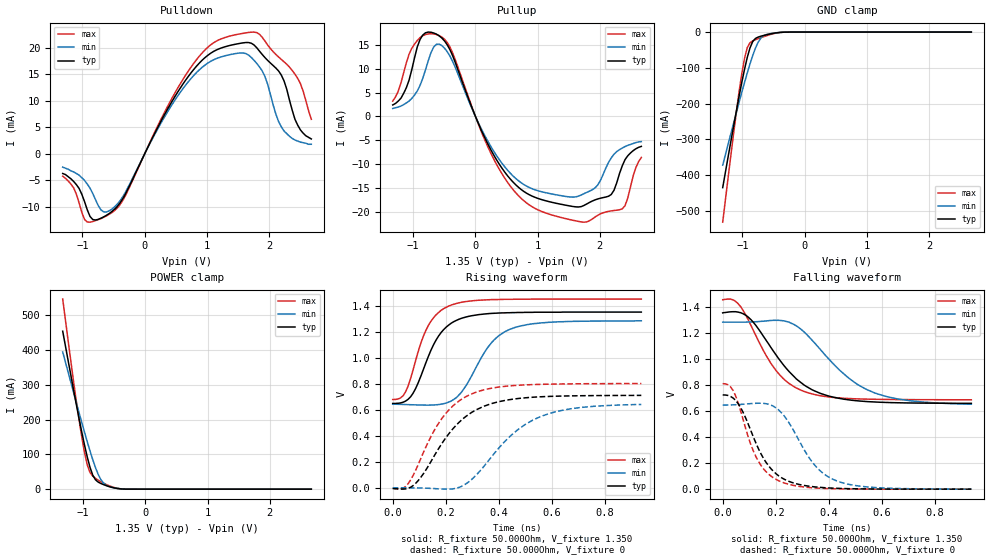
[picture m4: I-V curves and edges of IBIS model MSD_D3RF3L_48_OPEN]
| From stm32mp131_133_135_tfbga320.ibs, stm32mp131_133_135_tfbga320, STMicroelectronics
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[Model] MSD_D3RF3L_48_OPEN
Model_type   I/O
C_comp 2.572pF   2.485pF   2.698pF
Vinh = 810.000mV
Vinl = 540.000mV
Vmeas = 675.000mV
Vref = 675.000mV
[Model Spec]
Vinh   810.000mV   777.000mV   860.000mV
Vinl   540.000mV   507.000mV   590.000mV
Vmeas   675.000mV   642.000mV   725.000mV
Vref   675.000mV   642.000mV   725.000mV
[Receiver Thresholds]
Vth   =  0.675V
Vth_min  =  0.6615V
Vth_max  =  0.6885V
Vinh_ac  =  0.160V
Vinh_dc  =  0.090V
Vinl_ac  = -0.160V
Vinl_dc  = -0.090V
Tslew_ac =  5.000ns |Not specified, so set to high value
Threshold_sensitivity = 0.50
Reference_supply Pullup_ref
[Temperature Range]   25.000   125.000   -40.000
[Voltage Range]   1.350V   1.283V   1.450V
[GND Clamp Reference]   0.00V   0.00V   0.00V
[Pulldown Reference]   0.00V   0.00V   0.00V
[POWER Clamp Reference]   1.350V   1.283V   1.450V
[Pullup Reference]   1.350V   1.283V   1.450V
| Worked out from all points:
|   slope of the pulldown table from 0 to 0.203 V, typ, clamps not added: 42.2 ohm
|   slope of the pullup table from 0 to 0.203 V, typ, clamps not added: 34.5 ohm
|   GND clamp passes 1 mA (typ) near -0.40 V on its own axis
|   POWER clamp passes 1 mA (typ) near -0.41 V on its own axis
|   rising waveform, R_fixture 50.000Ohm, V_fixture 1.350: 20-80 % time 97.6ps typ, 120ps min, 83.7ps max; typ from 0.648 V to 1.35 V
|   rising waveform, R_fixture 50.000Ohm, V_fixture 0: 20-80 % time 163ps typ, 193ps min, 142ps max; typ from -0.004 V to 0.71 V
|   falling waveform, R_fixture 50.000Ohm, V_fixture 1.350: 20-80 % time 168ps typ, 200ps min, 137ps max; typ from 1.35 V to 0.659 V
|   falling waveform, R_fixture 50.000Ohm, V_fixture 0: 20-80 % time 108ps typ, 126ps min, 91.4ps max; typ from 0.723 V to 0 V
[GND Clamp]
-1.318V   -435mA     -372.2mA   -531.7mA
-1.142V   -262.4mA   -254.2mA   -282.5mA
-1.055V   -179.8mA   -196.6mA   -167.2mA
-1.011V   -140.5mA   -168.4mA   -116mA
-966.7mV  -103.7mA   -140.9mA   -72.98mA
-922.7mV  -70.73mA   -114.2mA   -43.23mA
-878.8mV  -44.02mA   -88.84mA   -29.72mA
-790.9mV  -17.74mA   -44.62mA   -21.37mA
-703mV    -11.46mA   -16.55mA   -15.5mA
-527.3mV  -4.197mA   -3.553mA   -5.598mA
-263.6mV  -40.6uA    -78.9uA    -28.72uA
2.68V     28.25nA    782nA      4.355nA
[Power Clamp]
-1.33V    454.4mA    394.7mA    546.8mA
-1.111V   243.5mA    248.7mA    252.9mA
-1.023V   163.7mA    191.5mA    149.8mA
-978.8mV  126.5mA    163.6mA    105.2mA
-934.9mV  92.34mA    136.2mA    69.61mA
-890.9mV  62.88mA    109.8mA    47.89mA
-847mV    40.47mA    84.8mA     37.29mA
-803mV    27.03mA    61.92mA    31.1mA
-715.1mV  16.21mA    27.03mA    21.42mA
-671.2mV  12.92mA    16.88mA    17.18mA
-407.6mV  989.1uA    1.283mA    1.2mA
2.668V    -48.24nA   -903.5nA   -4.583nA
[Pulldown]
-1.318V   -3.7mA     -2.5mA     -4.2mA
-1.055V   -6.5mA     -4mA       -9.2mA
-922.7mV  -10.54mA   -5.7mA     -12.83mA
-703mV    -12.11mA   -10.54mA   -12.18mA
-483.3mV  -10.4mA    -9.969mA   -10.66mA
790.9mV   15.9mA     14.77mA    17.06mA
1.582V    20.88mA    18.98mA    22.67mA
1.889V    18.72mA    15.62mA    21.96mA
2.197V    14.83mA    5.1mA      17.77mA
2.329V    10.1mA     3.3mA      16.32mA
2.461V    5.4mA      2.4mA      14.2mA
2.68V     2.8mA      1.8mA      6.5mA
[Pullup]
-1.33V    2.4mA      1.652mA    3.207mA
-1.023V   9.8mA      3.767mA    14.3mA
-890.9mV  16.12mA    6.477mA    16.51mA
-715.1mV  17.65mA    13.35mA    17.34mA
-451.5mV  14.98mA    13.54mA    15.46mA
295.4mV   -8.125mA   -7.33mA    -8.964mA
910.6mV   -16.72mA   -15.17mA   -18.95mA
1.702V    -18.92mA   -16.49mA   -22.14mA
1.965V    -17.33mA   -14.42mA   -20.77mA
2.185V    -16.38mA   -8.694mA   -19.82mA
2.361V    -10.4mA    -6.643mA   -19.39mA
2.668V    -6.3mA     -5.3mA     -8.621mA
[Ramp]
R_load=50.000Ohm
dV/dt_r   421.110mV/131.500ps  384.659mV/159.000ps  469.710mV/113.000ps
dV/dt_f   421.110mV/139.000ps  384.628mV/166.500ps  469.710mV/115.500ps
[Rising waveform]
R_fixture=50.000Ohm
V_fixture=1.350
V_fixture_min=1.283
V_fixture_max=1.450
0s        648.1mV    643.2mV    678.6mV
39ps      657.6mV    640.8mV    707.2mV
68ps      700.9mV    638.7mV    843.4mV
106ps     857.1mV    636.3mV    1.111V
135ps     1.012V     635.6mV    1.249V
211ps     1.25V      658.7mV    1.396V
259ps     1.302V     733.4mV    1.425V
374ps     1.34V      1.118V     1.446V
441ps     1.345V     1.217V     1.448V
938ps     1.35V      1.283V     1.45V
[Rising waveform]
R_fixture=50.000Ohm
V_fixture=0
0s        -4.082mV   715.5uV    -3.881mV
48ps      -7.901mV   807.6uV    9.802mV
87ps      35.87mV    91.83uV    137.1mV
183ps     333.3mV    -8.345mV   526.2mV
240ps     482.6mV    -2.622mV   651.4mV
298ps     579.8mV    64.92mV    721.7mV
451ps     680.6mV    411.2mV    784.9mV
556ps     699.4mV    546mV      794.9mV
710ps     707.7mV    617.6mV    799.6mV
938ps     710.4mV    640.6mV    801.1mV
[Falling waveform]
R_fixture=50.000Ohm
V_fixture=1.350
V_fixture_min=1.283
V_fixture_max=1.450
0s        1.353V     1.282V     1.454V
48ps      1.362V     1.282V     1.442V
96ps      1.321V     1.283V     1.301V
154ps     1.172V     1.289V     1.062V
202ps     1.028V     1.296V     908.6mV
298ps     813.6mV    1.223V     757.2mV
441ps     696.3mV    913.6mV    700mV
547ps     671.9mV    761.3mV    690.9mV
700ps     661.7mV    680.5mV    687.3mV
938ps     658.6mV    652.1mV    685.9mV
[Falling waveform]
R_fixture=50.000Ohm
V_fixture=0
0s        723.3mV    644.9mV    809.4mV
48ps      682.8mV    648mV      719.4mV
106ps     449.8mV    656.6mV    343mV
135ps     309.9mV    659.8mV    213mV
173ps     179.5mV    651.3mV    115.5mV
221ps     89.09mV    587.5mV    56.09mV
345ps     18.01mV    189.3mV    9.714mV
432ps     6.4mV      61.97mV    2.908mV
585ps     1.064mV    11.43mV    293.7uV
938ps     46.55uV    374uV      -860.8nV
